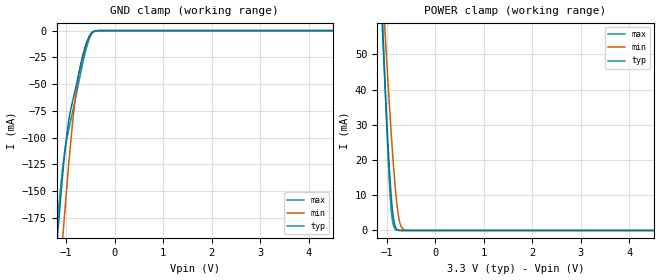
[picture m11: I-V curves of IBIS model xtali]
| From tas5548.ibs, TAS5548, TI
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|   xtrali Model
[Model]   xtali
Model_type   Input
Vinl = 0.8
Vinh = 2
|   typ   min   max
C_comp   1.067pF   1.052pF   1.078pF
[Voltage Range]   3.3   3   3.6
[Temperature Range]   27   125   0
[Power Clamp Reference]   3.3   3   3.6
[GND Clamp Reference]   -0   -0   -0
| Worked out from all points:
|   GND clamp passes 1 mA (typ) near -0.45 V on its own axis
|   POWER clamp passes 1 mA (typ) near -0.83 V on its own axis
[GND Clamp]
|   Voltage   I(typ)   I(min)   I(max)
-3.3V     -1.492A    -1.526A    -1.484A
-1.201V   -204.9mA   -269.1mA   -191.3mA
-1.162V   -182.3mA   -245.7mA   -169.9mA
-1.063V   -129.6mA   -187.9mA   -124.1mA
-1.003V   -103mA     -154.5mA   -104.9mA
-943.8mV  -82.82mA   -122.7mA   -91.24mA
-844.8mV  -61.35mA   -75.77mA   -71.27mA
-765.6mV  -45.4mA    -47.16mA   -53.66mA
-607.2mV  -15.41mA   -14.87mA   -20.16mA
-508.2mV  -3.929mA   -4.497mA   -5.725mA
-429mV    -573.9uA   -1.027mA   -994.6uA
6.58V     0A         0A         0A
[POWER Clamp]
|   Voltage   I(typ)   I(min)   I(max)
-3.3V     793.8mA    662.2mA    993.4mA
-1.102V   59.91mA    72mA       65.2mA
-1.063V   48.18mA    62.33mA    50.53mA
-1.043V   42.46mA    57.57mA    43.44mA
-983.4mV  26.22mA    43.63mA    23.7mA
-924mV    12.36mA    30.47mA    8.403mA
-904.2mV  8.669mA    26.33mA    5.043mA
-864.6mV  3.394mA    18.58mA    1.384mA
-805.2mV  502.5uA    8.947mA    138.3uA
-726mV    27.98uA    1.884mA    5.145uA
-587.4mV  132nA      48.55uA    3.361nA
6.58V     0A         0A         0A
